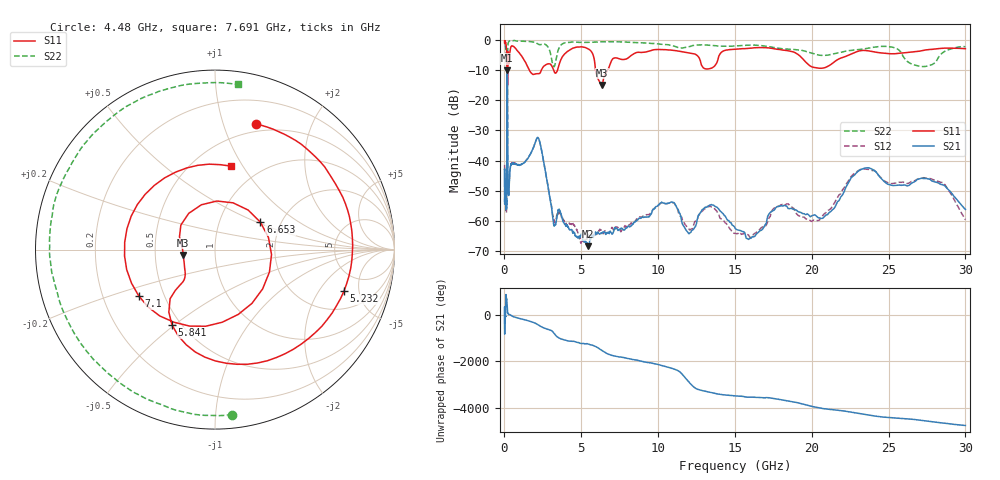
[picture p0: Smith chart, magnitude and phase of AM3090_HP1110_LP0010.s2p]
! Date/Time: Thu, Feb 28, 2019 2:08 PM
! Network Analyzer: Agilent Technologies E8364B Rev: A.07.50.67
! Sweep from 0.010 to 30.000 GHz, 1601 Points, Sweep Type: LOG
! Power Supply: 5.023 V, 0.002 A
# Hz S DB R 50
!freq MagS11 AngS11 MagS21 AngS21 MagS12 AngS12 MagS22 AngS22
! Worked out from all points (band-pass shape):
!   1601 points, 10 MHz to 30 GHz, reference 50 ohm
!   highest |S21| = -10.00 dB at 180.3 MHz (marker M1); lowest = -68.4 dB at 5.419 GHz (marker M2)
!   |S21| within 3 dB of the highest: 169.5 MHz to 193.1 MHz (23.67 MHz wide, 13.1 % of centre)
!   lowest |S11| = -14.9 dB at 6.328 GHz (marker M3), VSWR 1.44, Z = 34.9 - j2.19 ohm
!   |S11| at or under -10 dB: 1.619 GHz to 2.4 GHz (780.7 MHz wide, 38.9 % of centre); 3.201 GHz to 3.452 GHz (251.3 MHz wide, 7.55 % of centre); 5.931 GHz to 6.72 GHz (789.1 MHz wide, 12.5 % of centre)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
!   |S22| runs from -21.8 to -0.2 dB; largest |S21 - S12| = 0.01
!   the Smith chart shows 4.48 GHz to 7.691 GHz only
!   S11 on the Smith chart (normalised r, x): 4.48 GHz: 0.42, +1.29; 5.232 GHz: 3.24, -3.48; 5.841 GHz: 0.45, -0.49; 6.653 GHz: 1.57, +0.53; 7.1 GHz: 0.36, -0.25; 7.691 GHz: 0.74, +0.89
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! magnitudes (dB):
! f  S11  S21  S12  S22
! 10 MHz  -0.2  -48.5  -41.4  -0.5
! 38.04 MHz  -0.3  -51.5  -50.9  -1.1
! 144.7 MHz  -4.5  -49.6  -48.1  -8.7
! 165.6 MHz  -10.3  -16.3  -16.3  -14.0
! 180.3 MHz  -12.4  -10.0  -10.0  -21.4
! 231.6 MHz  -4.1  -50.2  -50.5  -1.4
! 550.5 MHz  -2.1  -40.7  -40.8  -0.3
! 2.084 GHz  -11.2  -32.9  -32.9  -1.0
! 3.22 GHz  -10.3  -61.4  -59.1  -8.9
! 4.48 GHz  -2.7  -63.5  -61.1  -0.7
! 5.232 GHz  -2.4  -67.0  -66.9  -0.8
! 5.419 GHz  -2.9  -68.4  -64.2  -0.8
! 5.841 GHz  -6.3  -64.7  -63.6  -0.7
! 6.328 GHz  -14.9  -64.0  -63.6  -0.6
! 6.653 GHz  -10.6  -63.8  -64.0  -0.6
! 7.1 GHz  -6.1  -63.6  -63.1  -0.6
! 7.691 GHz  -6.5  -62.6  -62.8  -0.6
! 7.926 GHz  -6.3  -62.4  -62.0  -0.7
! 10.65 GHz  -3.3  -54.2  -54.1  -1.6
! 16.21 GHz  -2.6  -65.3  -64.4  -1.7
! 23.48 GHz  -3.5  -42.5  -42.8  -2.9
! 30 GHz  -2.9  -56.2  -59.6  -2.2
